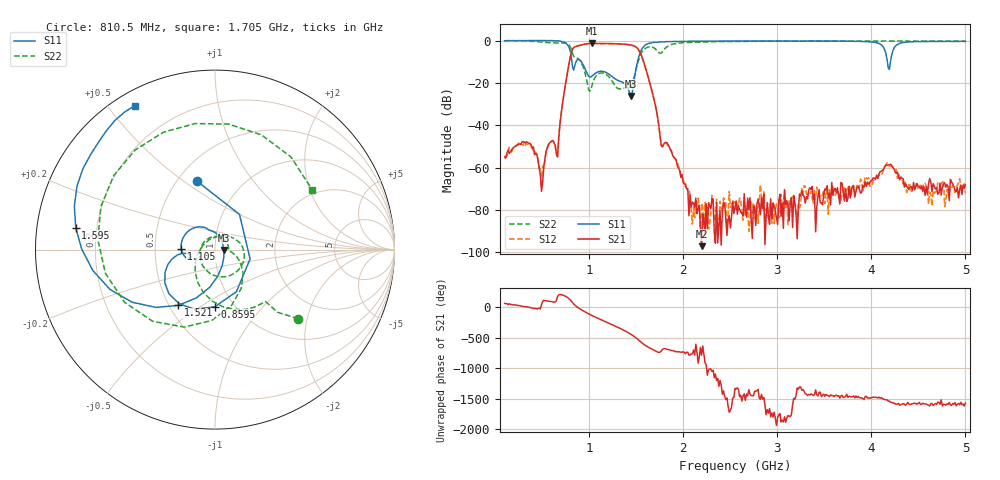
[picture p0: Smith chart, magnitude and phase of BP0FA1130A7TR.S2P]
! s2p File.  Ports: 1,3
# MHz S DB R 50
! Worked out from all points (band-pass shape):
!   401 points, 100 MHz to 5 GHz, reference 50 ohm
!   highest |S21| = -1.28 dB at 1.031 GHz (marker M1); lowest = -97.0 dB at 2.195 GHz (marker M2)
!   |S21| within 3 dB of the highest: 820.6 MHz to 1.524 GHz (703.1 MHz wide, 60 % of centre)
!   lowest |S11| = -26.1 dB at 1.448 GHz (marker M3), VSWR 1.10, Z = 55.2 - j0.184 ohm
!   |S11| at or under -10 dB: 816 MHz to 859.1 MHz (43.07 MHz wide, 5.14 % of centre); 916.5 MHz to 1.513 GHz (596.8 MHz wide, 49.1 % of centre); 4.171 GHz to 4.203 GHz (32.43 MHz wide, 0.775 % of centre)
!   |S22| runs from -23.9 to 0.0 dB; largest |S21 - S12| = 0.0035
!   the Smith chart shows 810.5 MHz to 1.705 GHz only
!   S11 on the Smith chart (normalised r, x): 810.5 MHz: 0.62, +0.56; 859.5 MHz: 0.82, -0.58; 1.105 GHz: 0.68, +0.01; 1.521 GHz: 0.56, -0.40; 1.595 GHz: 0.12, +0.08; 1.705 GHz: 0.06, +0.59
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100  -0.03 -11.1  -54.83 66.8  -55.48 67.0  -0.04 -33.6
296  0.04 -34.7  -47.69 16.4  -49.41 19.3  -0.14 -108.2
492  0.07 -64.9  -71.14 42.5  -68.96 74.5  -0.66 157.8
663.5  -0.06 -108.4  -54.92 -179.2  -53.80 -169.6  -1.11 66.8
810.5  -8.03 105.0  -5.47 101.4  -5.47 101.4  -4.41 -39.7
859.5  -9.94 -90.1  -2.67 21.7  -2.68 21.8  -8.02 -49.4
920.75  -10.27 -155.4  -1.93 -42.1  -1.93 -42.0  -10.85 -93.1
1031  -16.64 -159.4  -1.28 -133.6  -1.30 -133.7  -20.83 58.8
1104.5  -14.51 178.6  -1.33 173.9  -1.35 174.0  -15.44 -14.7
1251.5  -17.21 116.0  -1.39 73.2  -1.38 73.3  -19.68 -139.3
1447.5  -26.14 -1.9  -2.08 -83.9  -2.08 -83.9  -21.53 -6.7
1521  -8.60 -123.3  -4.10 -168.8  -4.08 -168.9  -9.72 -73.9
1594.5  -2.10 171.2  -12.29 100.1  -12.30 99.9  -3.68 175.1
1704.75  -0.74 119.1  -30.83 5.9  -30.79 5.9  -3.93 31.4
1741.5  -0.62 109.5  -40.63 -16.2  -40.85 -16.8  -5.65 -44.6
1815  -0.47 93.5  -48.01 39.6  -48.23 39.4  -3.27 161.0
1925.25  -0.36 75.7  -56.43 -1.6  -56.91 -3.8  -1.28 80.9
2194.75  -0.21 50.6  -97.04 -63.7  -76.77 -155.2  -0.58 7.0
2550  -0.15 31.6  -78.67 114.3  -76.16 94.8  -0.34 -40.4
3370.75  -0.14 6.6  -68.82 11.1  -74.02 -14.4  -0.14 -91.6
4191.5  -13.59 4.4  -58.60 -95.3  -59.25 -91.7  -0.19 -118.3
5000  -0.32 -35.2  -67.95 -129.9  -72.09 -179.4  -0.18 -146.5
